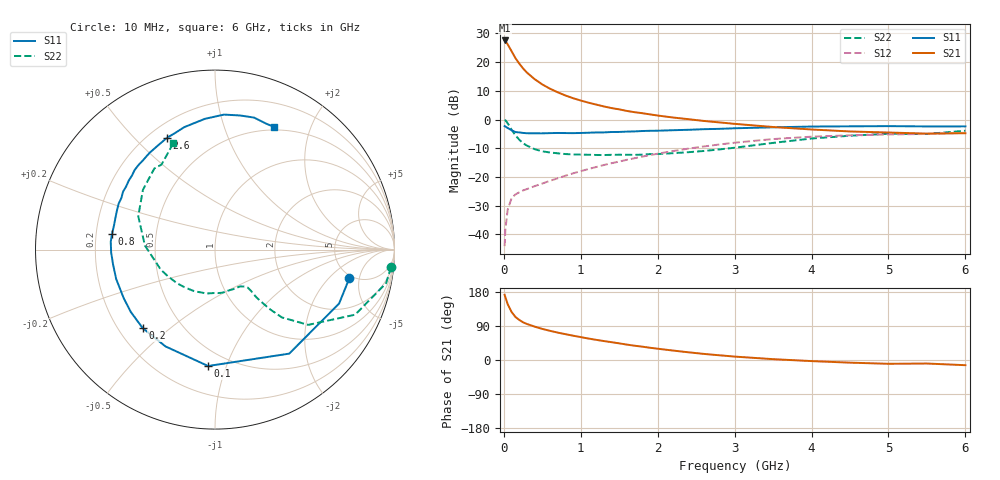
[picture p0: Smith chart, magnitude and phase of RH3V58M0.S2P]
! SIEMENS Small Signal Semiconductors
! BFR106
! Si NPN RF Bipolar Junction Transistor in SOT23
! VCE = 3.5 V  IC = 8 mA
! Common Emitter S-Parameters:  August  1996
# GHz  S  MA  R  50
!  f  S11  S21  S12  S22
! GHz  MAG  ANG  MAG  ANG  MAG  ANG  MAG  ANG
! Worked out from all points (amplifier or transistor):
!   36 points, 10 MHz to 6 GHz, reference 50 ohm
!   highest |S21| = 27.6 dB at 10 MHz (marker M1)
!   |S21| within 3 dB of that: start of sweep to 84.75 MHz
!   unconditionally stable (mu >= 1): 522.6 MHz to 2.077 GHz; 5.041 GHz to end of sweep
!   at 250 MHz: K = 0.64, MSG = 21.3 dB, |S12| = -24.7 dB
!   at 1.4 GHz: K = 1.11, MAG = 7.6 dB, |S12| = -15.2 dB
!   at 6 GHz: K = 1.01, MAG = -0.8 dB, |S12| = -4.6 dB
!   S11 on the Smith chart (normalised r, x): 10 MHz: 4.65, -3.60; 100 MHz: 0.39, -0.87; 200 MHz: 0.30, -0.40; 800 MHz: 0.27, +0.07; 2.6 GHz: 0.27, +0.63; 6 GHz: 0.46, +1.50
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0.01  0.7652 -12.1  23.86 172.0  0.0062 85.5  0.9859 -5.7
0.02  0.754 -23.5  23.25 165.8  0.0121 78.9  0.9715 -11.1
0.05  0.712 -54.5  20.41 147.3  0.0269 65.8  0.861 -24.9
0.1  0.6497 -93.4  15.55 127.0  0.0423 51.9  0.6677 -38.9
0.15  0.6058 -117.1  11.78 113.7  0.0494 45.0  0.5306 -45.4
0.2  0.5946 -132.7  9.455 105.8  0.0538 43.7  0.4459 -47.5
0.25  0.5837 -143.5  7.764 99.4  0.0581 43.5  0.3852 -48.5
0.3  0.5761 -152.1  6.573 95.1  0.0613 44.7  0.351 -49.1
0.4  0.5744 -163.5  5.052 88.1  0.0689 47.5  0.3044 -48.9
0.5  0.5739 -171.7  4.083 82.0  0.0765 50.5  0.2785 -49.3
0.6  0.5789 -178.5  3.442 77.0  0.0855 53.1  0.2662 -50.6
0.7  0.5825 175.6  2.981 72.3  0.0944 55.4  0.2577 -52.9
0.8  0.5803 171.4  2.624 68.2  0.1047 56.9  0.25 -55.1
1.1  0.5883 158.2  1.965 56.6  0.137 60.0  0.2429 -65.0
1.3  0.5956 151.1  1.689 50.0  0.1609 60.5  0.2401 -72.5
1.6  0.6154 141.3  1.409 40.6  0.1986 59.9  0.243 -85.9
2.2  0.6507 124.1  1.083 24.9  0.2821 54.8  0.2589 -116.2
2.6  0.6781 113.2  0.944 16.1  0.339 49.3  0.2827 -138.5
3.5  0.7308 94.4  0.74 2.2  0.4564 34.2  0.3911 176.7
4.5  0.7604 79.3  0.619 -7.0  0.5302 16.3  0.5218 140.3
5.5  0.7574 67.9  0.568 -9.3  0.5592 5.0  0.5594 122.2
6  0.7589 64.1  0.577 -13.7  0.5875 -2.7  0.6374 111.3
